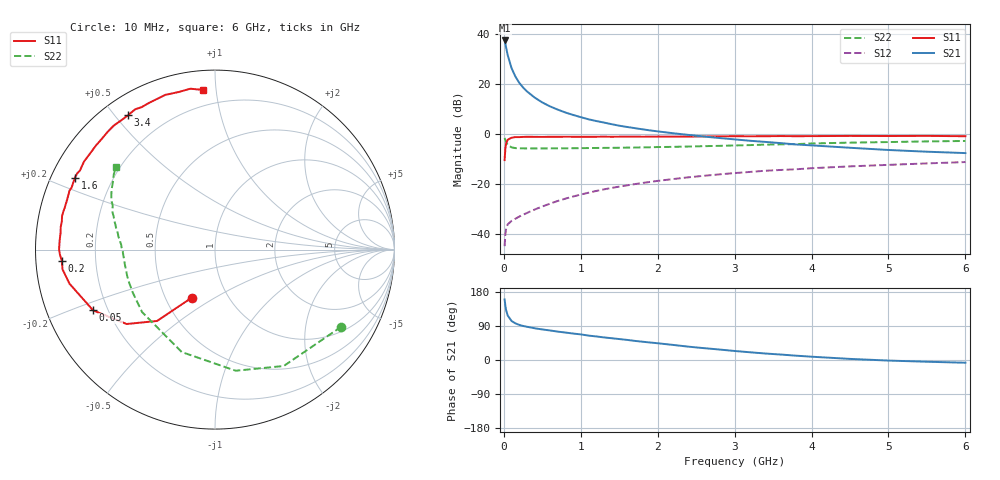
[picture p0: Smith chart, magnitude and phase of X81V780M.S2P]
! SIEMENS Small Signal Semiconductors
! BFP136W
! Si NPN RF Bipolar Junction Transistor in SOT343
! VCE = 1.75 V  IC = 80 mA
! Common Emitter S-Parameters:  September  1994
# GHz  S  MA  R  50
!  f  S11  S21  S12  S22
! GHz  MAG  ANG  MAG  ANG  MAG  ANG  MAG  ANG
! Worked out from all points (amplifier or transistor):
!   40 points, 10 MHz to 6 GHz, reference 50 ohm
!   highest |S21| = 37.2 dB at 10 MHz (marker M1)
!   |S21| within 3 dB of that: start of sweep to 30.76 MHz
!   unconditionally stable (mu >= 1): 490.7 MHz to 2.881 GHz
!   at 200 MHz: K = 0.67, MSG = 26.7 dB, |S12| = -33.1 dB
!   at 1.5 GHz: K = 1.11, MAG = 10.1 dB, |S12| = -21.1 dB
!   at 6 GHz: K = 0.98, MSG = 1.8 dB, |S12| = -11.3 dB
!   S11 on the Smith chart (normalised r, x): 10 MHz: 0.68, -0.40; 50 MHz: 0.14, -0.23; 200 MHz: 0.08, -0.04; 1.6 GHz: 0.07, +0.24; 3.4 GHz: 0.07, +0.54; 6 GHz: 0.11, +0.92
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0.01  0.2977 -115.8  72.8 159.8  0.0057 69.9  0.8245 -31.4
0.02  0.5124 -129.1  62.25 143.2  0.0099 58.9  0.7532 -59.4
0.03  0.6437 -139.9  52.22 131.4  0.0128 47.6  0.6847 -80.3
0.05  0.7587 -153.5  37.08 117.4  0.0155 38.1  0.6 -108.0
0.1  0.8325 -166.8  20.41 103.0  0.0182 34.9  0.535 -139.4
0.15  0.8565 -172.6  13.88 96.7  0.0201 37.8  0.5172 -152.3
0.2  0.8561 -175.8  10.41 92.7  0.0222 39.6  0.5125 -159.2
0.25  0.8651 -178.4  8.396 89.8  0.0242 43.5  0.5109 -163.6
0.3  0.8687 179.9  7.019 87.7  0.0262 45.9  0.5086 -166.6
0.4  0.867 176.4  5.281 83.8  0.0307 51.1  0.5091 -170.6
0.5  0.8653 173.9  4.213 80.6  0.0353 54.2  0.509 -173.3
0.6  0.8685 171.7  3.517 78.0  0.0403 56.8  0.5103 -175.0
0.7  0.8682 169.4  3.032 74.9  0.0455 58.8  0.5119 -176.3
0.9  0.871 165.9  2.374 69.8  0.0558 60.1  0.5139 -178.8
1.1  0.8694 161.7  1.944 64.4  0.0665 60.9  0.518 179.6
1.6  0.8769 152.9  1.367 53.1  0.0932 59.5  0.5288 175.6
2.2  0.8781 142.8  1.024 39.8  0.1246 55.3  0.547 171.0
3.2  0.8897 125.8  0.724 20.4  0.1729 45.7  0.5933 162.0
3.4  0.8919 122.8  0.687 17.1  0.1826 43.6  0.6065 160.2
4.5  0.9054 107.8  0.525 2.9  0.2232 33.2  0.6647 150.2
5.5  0.9068 98.7  0.438 -4.6  0.2559 25.3  0.7032 143.3
6  0.8919 94.3  0.411 -7.2  0.2722 20.8  0.7175 140.3
